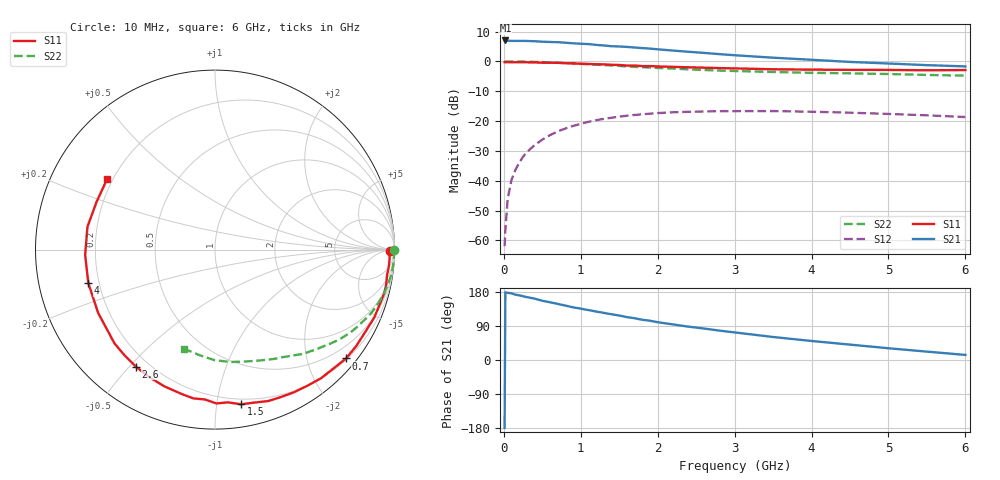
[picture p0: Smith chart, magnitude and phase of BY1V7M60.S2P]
! SIEMENS Small Signal Semiconductors
! BFY420
! Si NPN RF SIEGET Grounded Emitter Transistor in MICRO-X
! VCE = 1.75 V  IC = 0.6 mA
! Common Emitter S-Parameters:  October  1996
# GHz  S  MA  R  50
!  f  S11  S21  S12  S22
! GHz  MAG  ANG  MAG  ANG  MAG  ANG  MAG  ANG
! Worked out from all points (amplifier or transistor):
!   36 points, 10 MHz to 6 GHz, reference 50 ohm
!   highest |S21| = 7.1 dB at 20 MHz (marker M1)
!   |S21| within 3 dB of that: start of sweep to 2.012 GHz
!   unconditionally stable (mu >= 1): 4.746 GHz to end of sweep
!   at 250 MHz: K = 0.03, MSG = 19.4 dB, |S12| = -31.9 dB
!   at 1.4 GHz: K = 0.19, MSG = 12.0 dB, |S12| = -18.9 dB
!   at 6 GHz: K = 1.39, MAG = 4.8 dB, |S12| = -18.6 dB
!   S11 on the Smith chart (normalised r, x): 10 MHz: 68, -29; 700 MHz: 0.23, -2.75; 1.5 GHz: 0.16, -1.17; 2.6 GHz: 0.15, -0.52; 4 GHz: 0.16, -0.13; 6 GHz: 0.18, +0.29
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0.01  0.9754 -0.6  2.251 -179.2  0.0008 98.7  1 -0.2
0.02  0.972 -1.2  2.252 178.8  0.0015 79.5  0.9961 -0.6
0.05  0.9742 -3.0  2.226 177.3  0.005 86.9  0.998 -1.4
0.1  0.9729 -5.8  2.214 175.9  0.0104 86.5  0.9971 -2.8
0.15  0.9689 -8.6  2.212 172.3  0.0152 83.6  0.9965 -4.3
0.25  0.9738 -14.5  2.212 168.3  0.0254 80.6  0.9938 -7.1
0.4  0.9649 -23.0  2.186 161.9  0.0396 75.4  0.9833 -11.4
0.5  0.9548 -28.6  2.145 156.3  0.049 72.1  0.9743 -14.1
0.7  0.9491 -39.7  2.107 148.0  0.0672 65.3  0.9527 -19.3
0.9  0.9288 -50.5  2.018 139.0  0.083 57.9  0.9258 -24.3
1.1  0.9086 -61.0  1.957 131.7  0.0974 51.6  0.899 -29.0
1.4  0.8799 -75.7  1.803 120.7  0.1139 42.8  0.8577 -35.4
1.5  0.8739 -80.4  1.786 117.4  0.1188 39.7  0.8425 -37.4
1.8  0.8368 -93.9  1.677 106.2  0.1301 32.2  0.8017 -42.9
2.2  0.8124 -110.3  1.524 93.9  0.1407 23.0  0.761 -49.8
2.6  0.787 -124.0  1.393 83.1  0.1451 15.4  0.72 -55.7
3  0.7659 -137.0  1.273 72.8  0.1469 9.0  0.6929 -61.5
3.5  0.7406 -151.5  1.157 60.7  0.1474 2.1  0.6666 -67.9
4  0.73 -165.2  1.068 50.2  0.1437 -3.6  0.646 -74.8
4.5  0.724 -177.7  0.983 40.6  0.1385 -8.5  0.6325 -81.9
5.5  0.7114 158.1  0.868 22.1  0.1251 -14.3  0.5946 -98.3
6  0.7187 146.6  0.827 13.4  0.117 -14.7  0.5785 -107.5
